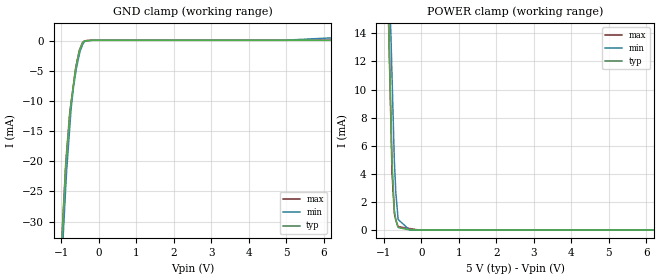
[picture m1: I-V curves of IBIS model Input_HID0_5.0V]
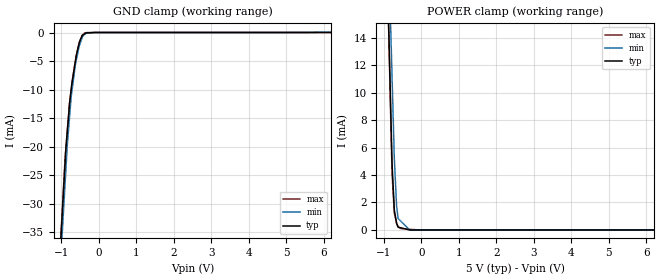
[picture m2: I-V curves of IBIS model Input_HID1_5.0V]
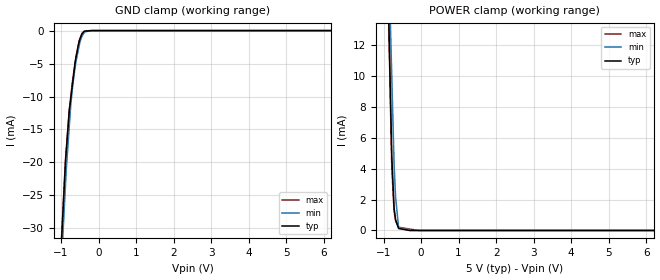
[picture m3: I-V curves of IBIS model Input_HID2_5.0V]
[IBIS Ver]   4.0
[Comment Char] |_char
[File Name]   pcm2903c.ibs
[File Rev]   1.0
[Source]
[Date]   9-15-2011
[Notes]   Quality Check of this IBIS model: Model Passes IBIS Check
   Model parses into ICX IS. Simulation done with Hyperlynx.
   1. MIN TYP MAX information is based on Temprature and Voltage
   characteristics only.
   2. Please note that pins, DIN and DOUT, are not modeled as specified NCs.
[Disclaimer]
 This product is designed as an aid for customers of Texas Instruments.
 No warranties, either expressed or implied, with respect to this third
 party software (if any) or with respect to its fitness for any
 particular purpose is claimed by Texas Instruments or the author. The
 software (if any) is provided solely on an "as is" basis. The entire
 risk as to its quality and performance is with the customer
[Copyright] (C) Copyright 2011 Texas Instruments Incorporated.
   All rights reserved.
[Component] PCM2903C
[Manufacturer] TI
[Package]
| variable   typ   min   max
R_pkg  1.8006E-02  1.8006E-02  1.8006E-02
L_pkg  2.1607E-09  2.1607E-09  2.1607E-09
C_pkg  6.0021E-13  6.0021E-13  6.0021E-13
[Pin] signal_name  model_name  R_pin  L_pin C_pin
1   D+   USB_5.0V   1.9723E-02  2.3076E-09  5.4618E-13
2   D-   USB_5.0V   1.8868E-02  2.2076E-09  5.2250E-13
3   Vbus   POWER   1.8028E-02  2.1092E-09  4.9923E-13
4   DGNDU   GND   1.7205E-02  2.0129E-09  4.7644E-13
5   HID0   Input_HID0_5.0V   1.6401E-02  1.9189E-09  4.5419E-13
6   HID1   Input_HID1_5.0V   1.5620E-02  1.8276E-09  4.3257E-13
7   HID2   Input_HID2_5.0V   1.4866E-02  1.7393E-09  4.1168E-13
8   SEL0   Input_SEL0_5.0V   1.4866E-02  1.7393E-09  4.1168E-13
9   SEL1   Input_SEL1_5.0V   1.5620E-02  1.8276E-09  4.3257E-13
10  VCCCI   POWER   1.6401E-02  1.9189E-09  4.5419E-13
11  AGNDC   GND   1.7205E-02  2.0129E-09  4.7644E-13
12  VinL   Analog_In   1.8028E-02  2.1092E-09  4.9923E-13
13  VinR   Analog_In   1.8868E-02  2.2076E-09  5.2250E-13
14  Vcom   POWER   1.9723E-02  2.3076E-09  5.4618E-13
15  VoutR   NC   1.9723E-02  2.3076E-09  5.4618E-13
16  VoutL   NC   1.8868E-02  2.2076E-09  5.2250E-13
17  VCCP1I  POWER   1.8028E-02  2.1092E-09  4.9923E-13
18  AGNDP   GND   1.7205E-02  2.0129E-09  4.7644E-13
19  VCCP2I  POWER   1.6401E-02  1.9189E-09  4.5419E-13
20  XTO   Output_XTO_5.0V   1.5620E-02  1.8276E-09  4.3257E-13
21  XTI   Input_XTI_5.0V   1.4866E-02  1.7393E-09  4.1168E-13
22  AGNDX   GND   1.4866E-02  1.7393E-09  4.1168E-13
23  VCCXI   POWER   1.5620E-02  1.8276E-09  4.3257E-13
24  DIN   NC   1.6401E-02  1.9189E-09  4.5419E-13
25  DOUT   NC   1.7205E-02  2.0129E-09  4.7644E-13
26  DGND   GND   1.8028E-02  2.1092E-09  4.9923E-13
27  VDDI   POWER   1.8868E-02  2.2076E-09  5.2250E-13
28  _SSPND  Output_SSPND_5.0V  1.9723E-02  2.3076E-09  5.4618E-13
| Models and submodels in the file (10): Input_HID0_5.0V (Input), Input_HID1_5.0V (Input), Input_HID2_5.0V (Input), Input_SEL0_5.0V (Input), Input_SEL1_5.0V (Input), Input_XTI_5.0V (Input), Analog_In (Input), Output_SSPND_5.0V (Output), Output_XTO_5.0V (Output), USB_5.0V (I/O)
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[Model] Input_HID0_5.0V
Model_type Input
Vinl  = 900.000mV
Vinh  = 2.52000V
C_comp  2.00000pF 2.00000pF 2.00000pF
| variable   typ   min   max
[Voltage Range]   5.00000V  4.50000V  5.50000V
[POWER Clamp Reference]  5.00000V  4.50000V  5.50000V
[GND Clamp Reference]   0.00000V  0.00000V  0.00000V
[Temperature Range]   25   85   -25
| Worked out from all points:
|   GND clamp passes 1 mA (typ) near -0.48 V on its own axis
|   POWER clamp passes 1 mA (typ) near -0.70 V on its own axis
[GND Clamp]
-5V       -516.7mA   -511.3mA   -516.9mA
-881.1mV  -20.69mA   -24.2mA    -20.2mA
-861mV    -19.12mA   -21.83mA   -18.62mA
-780.2mV  -12.77mA   -14.83mA   -12.28mA
-760.1mV  -11.19mA   -13.08mA   -11.31mA
-739.6mV  -10.26mA   -11.31mA   -10.32mA
-679mV    -7.53mA    -7.887mA   -7.391mA
-623.5mV  -5.02mA    -5.556mA   -4.707mA
-522mV    -1.726mA   -2.33mA    -1.604mA
-380.7mV  -26.86uA   -130.3uA   -17.92uA
4.936V    100.6uA    99.12uA    98.92uA
10V       100.6uA    1.685mA    98.92uA
[POWER Clamp]
-5V       474.9mA    423mA      493.3mA
-1.139V   44.73mA    45.92mA    45.58mA
-780.6mV  4.768mA    10.9mA     4.029mA
-719.7mV  1.418mA    4.948mA    1.152mA
-679.5mV  698.8uA    2.661mA    700.7uA
-618.7mV  176.3uA    747.4uA    239uA
-309.4mV  0A         0A         104.4uA
-38.05mV  0A         0A         0A
10V       0A         0A         0A
[Model] Input_HID1_5.0V
Model_type Input
Vinl  = 900.000mV
Vinh  = 2.52000V
C_comp  2.00000pF 2.00000pF 2.00000pF
| variable   typ   min   max
[Voltage Range]   5.00000V  4.50000V  5.50000V
[POWER Clamp Reference]  5.00000V  4.50000V  5.50000V
[GND Clamp Reference]   0.00000V  0.00000V  0.00000V
[Temperature Range]   25   85   -25
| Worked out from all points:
|   GND clamp passes 1 mA (typ) near -0.48 V on its own axis
|   POWER clamp passes 1 mA (typ) near -0.69 V on its own axis
[GND Clamp]
-5V       -510.3mA   -496.9mA   -522.5mA
-901.2mV  -22.99mA   -26.65mA   -22.17mA
-881mV    -20.59mA   -24.34mA   -20.53mA
-840.8mV  -17.32mA   -19.72mA   -17.24mA
-780.3mV  -12.41mA   -14.73mA   -12.3mA
-739.6mV  -10.11mA   -11.37mA   -10.11mA
-699.4mV  -8.132mA   -9.333mA   -7.946mA
-623.5mV  -4.932mA   -5.483mA   -4.858mA
-522.2mV  -1.708mA   -2.272mA   -1.631mA
-441.3mV  -400.7uA   -733uA     -386.5uA
-380.7mV  -169.7uA   -182.3uA   -3.574uA
10V       97.76uA    355.4uA    97.35uA
[POWER Clamp]
-5V       474mA      422.8mA    493.3mA
-1.099V   40.2mA     42.19mA    40.95mA
-780.5mV  4.815mA    11.13mA    4.078mA
-719.6mV  1.436mA    5.191mA    1.218mA
-659mV    474uA      1.719mA    485.8uA
-618.6mV  203.7uA    828.6uA    236.7uA
-549.4mV  158.1uA    643.2uA    104.4uA
-309.3mV  0A         0A         54.26uA
-30.65mV  0A         0A         0A
10V       0A         0A         0A
[Model] Input_HID2_5.0V
Model_type Input
Vinl  = 900.000mV
Vinh  = 2.52000V
C_comp  2.00000pF 2.00000pF 2.00000pF
| variable   typ   min   max
[Voltage Range]   5.00000V  4.50000V  5.50000V
[POWER Clamp Reference]  5.00000V  4.50000V  5.50000V
[GND Clamp Reference]   0.00000V  0.00000V  0.00000V
[Temperature Range]   25   85   -25
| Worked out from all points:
|   GND clamp passes 1 mA (typ) near -0.48 V on its own axis
|   POWER clamp passes 1 mA (typ) near -0.69 V on its own axis
[GND Clamp]
-5V       -490.3mA   -481mA     -486mA
-881mV    -19.91mA   -23.4mA    -19.55mA
-861mV    -18.36mA   -21.18mA   -18.05mA
-780.3mV  -12.13mA   -14.52mA   -12.03mA
-739.6mV  -10.21mA   -11.15mA   -9.921mA
-679mV    -7.345mA   -7.771mA   -7.012mA
-623.5mV  -4.729mA   -5.493mA   -4.778mA
-522.2mV  -1.738mA   -2.361mA   -1.576mA
-461.6mV  -676.1uA   -1mA       -654.5uA
-380.8mV  1.387uA    -238.4uA   -51.52uA
-180.2mV  86.27uA    97uA       85.92uA
10V       86.27uA    97uA       93.9uA
[POWER Clamp]
-5V       470.7mA    400.2mA    488.3mA
-1.119V   42.22mA    41.28mA    42.94mA
-780.5mV  4.808mA    9.951mA    4.088mA
-719.7mV  1.486mA    4.328mA    1.263mA
-679.5mV  696.9uA    2.177mA    629.7uA
-598.5mV  127uA      191.9uA    211.2uA
-299.3mV  0A         0A         93.9uA
-58.45mV  0A         0A         0A
10V       0A         0A         0A
